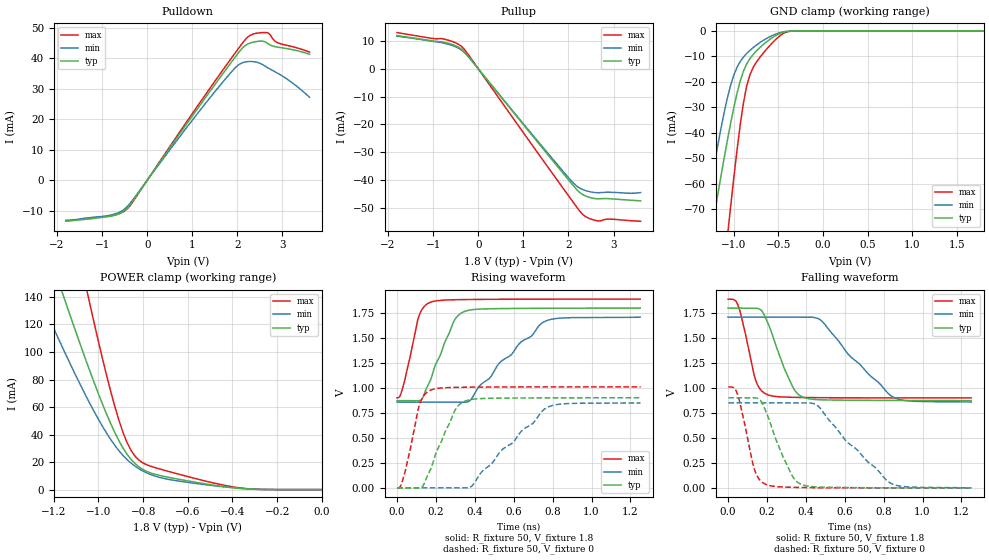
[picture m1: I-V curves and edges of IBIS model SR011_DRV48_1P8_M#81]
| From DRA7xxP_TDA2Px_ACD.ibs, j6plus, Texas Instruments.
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| Model based on original model for DDR_SEIOPB_V
|   Sub model SR011_DRV48_1P8
[model]   SR011_DRV48_1P8_M#81
|[Description]  [1.8V-I/O-X-X]
|   , ,
|[Input Load]
|[Output Drive]
|Voltage   1.8V
|Mode   I/O
Model_type   I/O
Polarity   Non-Inverting
Enable   Active-Low
Vinl =  0.775
Vinh =  1.025
Cref =  15.0000pF
Rref =  100.0000M
Vref =  0V
Vmeas =  0.9
C_comp   2p   2p   2p
[Model Spec]
Vinl   0.78   0.735   0.825
Vinh   1.02   0.975   1.065
[Receiver Thresholds]
Tslew_ac = 0.5n
Vth = 0.9
Vth_max = 0.945
Vth_min = 0.81
Vinh_ac = 0.2
Vinh_dc = 0.125
Vinl_ac = -0.2
Vinl_dc = -0.125
[Temperature Range]   25   125   -40
[Voltage Range]   1.8   1.71   1.89
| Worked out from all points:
|   slope of the pulldown table from 0 to 0.27 V, typ, clamps not added: 46.9 ohm
|   slope of the pullup table from 0 to 0.27 V, typ, clamps not added: 49.7 ohm
|   GND clamp passes 1 mA (typ) near -0.48 V on its own axis
|   POWER clamp passes 1 mA (typ) near -0.38 V on its own axis
|   rising waveform, R_fixture 50, V_fixture 1.8: 20-80 % time 113ps typ, 272ps min, 65.7ps max; typ from 0.874 V to 1.8 V
|   rising waveform, R_fixture 50, V_fixture 0: 20-80 % time 114ps typ, 272ps min, 65.7ps max; typ from 0 V to 0.903 V
|   falling waveform, R_fixture 50, V_fixture 1.8: 20-80 % time 108ps typ, 249ps min, 67.4ps max; typ from 1.8 V to 0.874 V
|   falling waveform, R_fixture 50, V_fixture 0: 20-80 % time 111ps typ, 255ps min, 66.8ps max; typ from 0.903 V to 0 V
[POWER_clamp]
-1.8V     464.6mA    344.4mA    740.8mA
-1.273V   197mA      143.3mA    314.4mA
-1.164V   144mA      104.2mA    229mA
-1.145V   135.3mA    97.86mA    215mA
-1.055V   93.25mA    67.59mA    146.5mA
-1.036V   85.18mA    61.89mA    133.3mA
-909.1mV  35.72mA    28.41mA    50.73mA
-872.7mV  25.87mA    21.94mA    34.5mA
-818.2mV  16.45mA    15.08mA    21.33mA
-690.9mV  9.084mA    7.592mA    13.42mA
-400mV    1.38mA     1.43mA     2.039mA
0V        227.3nA    761nA      1.176uA
[Pulldown]
-1.8V     -13.45mA   -13.11mA   -13.3mA
-818.2mV  -11.81mA   -11.44mA   -11.72mA
-600mV    -10.83mA   -10.36mA   -10.81mA
-436.4mV  -9.068mA   -8.512mA   -9.288mA
1.255V    26.38mA    24.53mA    27.32mA
1.855V    38.53mA    35.35mA    39.84mA
2.073V    42.76mA    38.34mA    44.25mA
2.291V    45.11mA    39mA       47.65mA
2.618V    45.4mA     37.45mA    48.49mA
2.727V    44.4mA     36.48mA    47.76mA
2.891V    43.71mA    35.16mA    45.15mA
3.6V      41.36mA    27.26mA    42.08mA
[Pullup]
-1.8V     11.9mA     11.66mA    12.97mA
-1.036V   10.04mA    9.888mA    10.91mA
-763.6mV  9.523mA    9.186mA    10.68mA
-490.9mV  8.144mA    7.787mA    9.204mA
-327.3mV  6.377mA    6.133mA    7.311mA
2.018V    -40.23mA   -39.43mA   -46mA
2.182V    -43.37mA   -42.12mA   -49.65mA
2.345V    -45.48mA   -43.6mA    -52.72mA
2.509V    -46.4mA    -44.3mA    -54.07mA
2.673V    -46.74mA   -44.55mA   -54.7mA
2.891V    -46.69mA   -44.38mA   -54.01mA
3.6V      -47.48mA   -44.49mA   -54.81mA
[GND_clamp]
-1.8V     -200.8mA   -187.9mA   -345.9mA
-1.327V   -95.75mA   -76.22mA   -171.1mA
-1.255V   -80.19mA   -60.47mA   -144.9mA
-1.218V   -72.53mA   -52.92mA   -131.9mA
-1.073V   -43.32mA   -26.59mA   -81.54mA
-1.036V   -36.61mA   -21.6mA    -69.55mA
-963.6mV  -24.61mA   -14.37mA   -47.01mA
-854.5mV  -12.98mA   -8.864mA   -21.66mA
-781.8mV  -9.263mA   -6.573mA   -14.36mA
-672.7mV  -5.498mA   -3.827mA   -8.897mA
-345.5mV  -48.81uA   -73.08uA   -79.37uA
1.8V      227.3nA    3.986uA    988nA
[Ramp]
dV/dt_f 0.55611077/0.10855036n 0.51147507/0.24923733n 0.59374363/67.398245p
dV/dt_r 0.54238355/0.1140021n 0.51210158/0.27305893n 0.60770805/65.780899p
R_load = 50
[Rising Waveform]
R_fixture = 50
V_fixture = 1.8
V_fixture_min = 1.71
V_fixture_max = 1.89
0s        873.8mV    858.6mV    901.7mV
16.25ps   873.7mV    858.6mV    923.3mV
35.86ps   873.2mV    858.6mV    1.046V
112.8ps   872.9mV    858.6mV    1.721V
170ps     1.068V     858.6mV    1.857V
291.1ps   1.663V     858.5mV    1.884V
350.7ps   1.769V     857.4mV    1.886V
529.2ps   1.795V     1.256V     1.889V
758.9ps   1.798V     1.666V     1.89V
1.25ns    1.8V       1.71V      1.89V
[Rising Waveform]
R_fixture = 50
V_fixture = 0
V_fixture_min = 0
V_fixture_max = 0
1.934ps   0V         0V         0V
19.14ps   0V         0V         21.72mV
39.11ps   0V         0V         142.8mV
116.3ps   0V         0V         836.1mV
172.4ps   184.3mV    0V         978.4mV
295.7ps   768.5mV    0V         1.006V
354.6ps   872.3mV    0V         1.008V
386.2ps   886.5mV    20.84mV    1.009V
775.7ps   901.2mV    808.4mV    1.011V
1.252ns   902.5mV    851.6mV    1.011V
[Falling Waveform]
R_fixture = 50
V_fixture = 1.8
V_fixture_min = 1.71
V_fixture_max = 1.89
0s        1.8V       1.71V      1.89V
49.92ps   1.8V       1.71V      1.836V
140.9ps   1.8V       1.71V      1.086V
200.2ps   1.67V      1.71V      935.3mV
328.9ps   1.026V     1.71V      907mV
388.6ps   906.2mV    1.711V     904.9mV
480.5ps   881.8mV    1.673V     903mV
623.2ps   877.5mV    1.327V     901.7mV
851.7ps   875.2mV    905.9mV    901mV
1.25ns    873.8mV    858.6mV    900.8mV
[Falling Waveform]
R_fixture = 50
V_fixture = 0
V_fixture_min = 0
V_fixture_max = 0
1.934ps   902.5mV    851.6mV    1.011V
45.1ps    902.7mV    851.6mV    957.2mV
135.4ps   902.7mV    851.6mV    187.7mV
195ps     762.7mV    851.6mV    34.21mV
322.4ps   148.5mV    851.5mV    5.678mV
380.7ps   32mV       851.8mV    3.428mV
464.1ps   8.185mV    818mV      0V
605.5ps   3.249mV    472.3mV    0V
840ps     0V         42.9mV     0V
1.252ns   0V         0V         0V
